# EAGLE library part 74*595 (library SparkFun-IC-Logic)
8-Bit Shift Register (Serial to Parallel) Datasheet SparkFun Products SparkFun Shift Register Breakout - 74HC595 (BOB-10680)
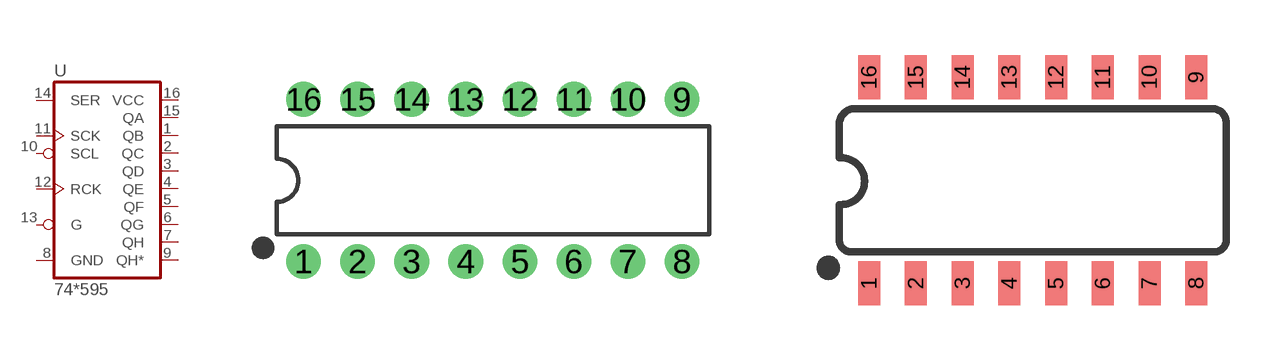
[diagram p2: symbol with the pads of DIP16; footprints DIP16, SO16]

Designator prefix U

## 74HC595N (PROD_ID: IC-13123; VALUE: SN74HC595N)  [DIP16]
1  QB  hiz
2  QC  hiz
3  QD  hiz
4  QE  hiz
5  QF  hiz
6  QG  hiz
7  QH  hiz
8  GND  pwr
9  QH*  hiz
10  SCL  in
11  SCK  in
12  RCK  in
13  G  in
14  SER  in
15  QA  hiz
16  VCC  pwr

## 74HC595D (PROD_ID: IC-07875; VALUE: SN74HC595D)  [SO16]
Pads as for DIP16

## 74LS595FK  [LCC20]
2  QB  hiz
3  QC  hiz
4  QD  hiz
5  QE  hiz
7  QF  hiz
8  QG  hiz
9  QH  hiz
10  GND  pwr
12  QH*  hiz
13  SCL  in
14  SCK  in
15  RCK  in
17  G  in
18  SER  in
19  QA  hiz
20  VCC  pwr

## 74595  [TSSOP16]
Pads as for DIP16

## Footprint DIP16 (pad centres in mm)
Dual In Line Package
drill 0.813 pad 1.626: 1 -8.89,-3.81; 2 -6.35,-3.81; 3 -3.81,-3.81; 4 -1.27,-3.81; 5 1.27,-3.81; 6 3.81,-3.81; 7 6.35,-3.81; 8 8.89,-3.81; 9 8.89,3.81; 10 6.35,3.81; 11 3.81,3.81; 12 1.27,3.81; 13 -1.27,3.81; 14 -3.81,3.81; 15 -6.35,3.81; 16 -8.89,3.81

## Footprint SO16 (pad centres in mm)
SOIC, 0.15 inch width
smd 0.6 x 1.2: 1 -4.445,-2.8; 2 -3.175,-2.8; 3 -1.905,-2.8; 4 -0.635,-2.8; 5 0.635,-2.8; 6 1.905,-2.8; 7 3.175,-2.8; 8 4.445,-2.8; 9 4.445,2.8; 10 3.175,2.8; 11 1.905,2.8; 12 0.635,2.8; 13 -0.635,2.8; 14 -1.905,2.8; 15 -3.175,2.8; 16 -4.445,2.8

## Footprint LCC20 (pad centres in mm)
Leadless Chip Carrier Ceramic Package
smd 0.8 x 3.4: 1 0,3.8
smd 0.8 x 2: 2 -1.27,4.5; 3 -2.54,4.5; 9 -2.54,-4.5; 10 -1.27,-4.5; 11 0,-4.5; 12 1.27,-4.5; 13 2.54,-4.5; 19 2.54,4.5; 20 1.27,4.5
smd 2 x 0.8: 4 -4.5,2.54; 5 -4.5,1.27; 6 -4.5,0; 7 -4.5,-1.27; 8 -4.5,-2.54; 14 4.5,-2.54; 15 4.5,-1.27; 16 4.5,0; 17 4.5,1.27; 18 4.5,2.54

## Footprint TSSOP16 (pad centres in mm)
TSOP16 thin small outline package
smd 0.4 x 1.6: 1 -2.225,-2.85; 2 -1.575,-2.85; 3 -0.925,-2.85; 4 -0.275,-2.85; 5 0.375,-2.85; 6 1.025,-2.85; 7 1.675,-2.85; 8 2.325,-2.85; 9 2.325,3.05; 10 1.675,3.05; 11 1.025,3.05; 12 0.375,3.05; 13 -0.275,3.05; 14 -0.925,3.05; 15 -1.575,3.05; 16 -2.225,3.05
